(* Logix 5000 AddOnInstructionDefinition export; software revision 16.04 *)

ADD_ON_INSTRUCTION AMCI_ANG1E_Encoder_Follower   (* revision 1.1, vendor AMCI, ExecuteEnableInFalse *)
// Revision note:
// Version 1.1 added the slot_axis number and the input parameters can now be tags or discrete values.
VAR_INPUT
   Axis_Status_Bits : INT; {required}
   slot_axis_number : INT; {required}
   Electronic_Gearing_Numerator : INT; {required}
   Electronic_Gearing_Denominator : INT; {required}
   Programmed_Speed : DINT; {required}
   Acceleration : INT; {required}
   Deceleration : INT; {required}
   jerk : INT;
END_VAR
VAR_IN_OUT
   AMCI_ANG1E_output_data : INT[10]; {required}
END_VAR
VAR_OUTPUT
   EN : BOOL; {visible}
   Encoder_Follower_Occurring : BOOL; {visible}
   ER : BOOL; {visible}
END_VAR
VAR
   Upper_Result_X_1000 : DINT;
   command_data_block : INT[10];
        [0]   // Command Bits MSW
        [1]   // Command Bits LSW
        [4]   // Upper Programmed Speed
        [5]   // Lower Programmed Speed
   index : INT;
END_VAR

ROUTINE EnableInFalse   (* ladder *)
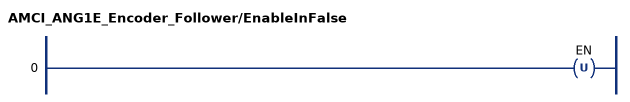
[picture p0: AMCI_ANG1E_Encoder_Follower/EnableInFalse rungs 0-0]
   0: OTU(EN);
END_ROUTINE

ROUTINE Logic   (* ladder *)
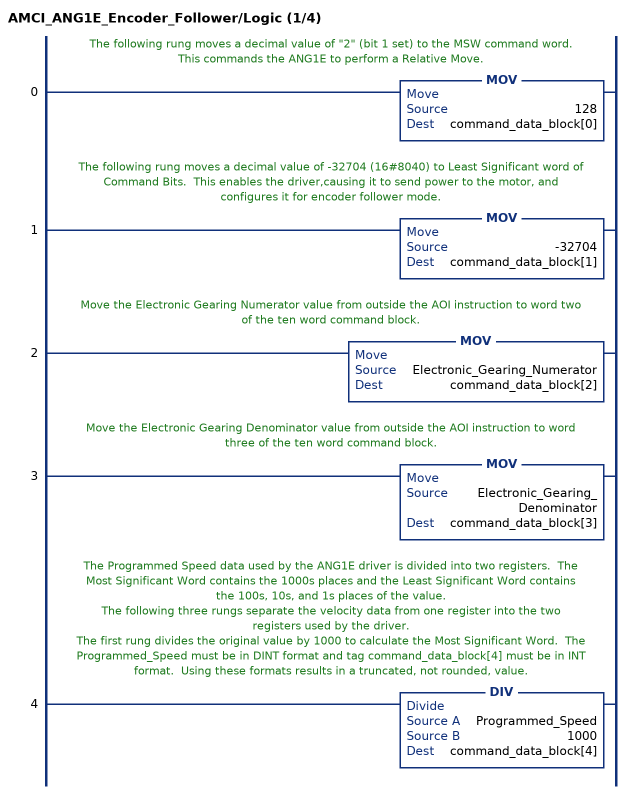
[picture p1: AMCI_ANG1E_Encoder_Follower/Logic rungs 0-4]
   // The following rung moves a decimal value of "2" (bit 1 set) to the MSW command word.  This commands the ANG1E to perform a Relative Move.
   0: MOV(128,command_data_block[0]);
   // The following rung moves a decimal value of -32704 (16#8040) to Least Significant word of Command Bits.  This enables the driver,causing it to send power to the motor, and configures it for encoder follower mode.
   1: MOV(-32704,command_data_block[1]);
   // Move the Electronic Gearing Numerator value from outside the AOI instruction to word two of the ten word command block.
   2: MOV(Electronic_Gearing_Numerator,command_data_block[2]);
   // Move the Electronic Gearing Denominator value from outside the AOI instruction to word three of the ten word command block.
   3: MOV(Electronic_Gearing_Denominator,command_data_block[3]);
   // The Programmed Speed data used by the ANG1E driver is divided into two registers.  The Most Significant Word contains the 1000s places and the Least Significant Word contains the 100s, 10s, and 1s places of the value.
   // The following three rungs separate the velocity data from one register into the two registers used by the driver.
   // The first rung divides the original value by 1000 to calculate the Most Significant Word.  The Programmed_Speed must be in DINT format and tag command_data_block[4] must be in INT format.  Using these formats results in a truncated, not rounded, value.
   4: DIV(Programmed_Speed,1000,command_data_block[4]);
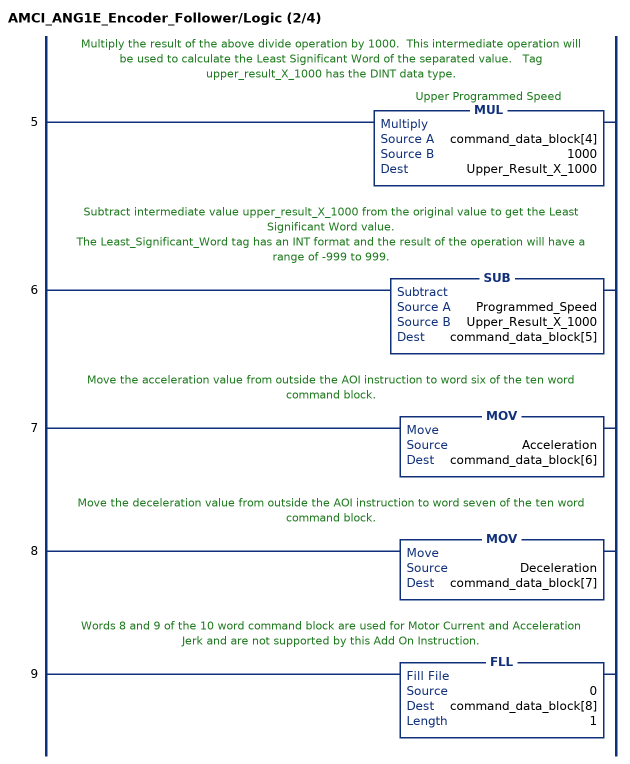
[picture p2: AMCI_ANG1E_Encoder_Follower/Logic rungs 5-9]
   // Multiply the result of the above divide operation by 1000.  This intermediate operation will be used to calculate the Least Significant Word of the separated value.   Tag upper_result_X_1000 has the DINT data type.
   5: MUL(command_data_block[4],1000,Upper_Result_X_1000);
   // Subtract intermediate value upper_result_X_1000 from the original value to get the Least Significant Word value.
   // The Least_Significant_Word tag has an INT format and the result of the operation will have a range of -999 to 999.
   6: SUB(Programmed_Speed,Upper_Result_X_1000,command_data_block[5]);
   // Move the acceleration value from outside the AOI instruction to word six of the ten word command block.
   7: MOV(Acceleration,command_data_block[6]);
   // Move the deceleration value from outside the AOI instruction to word seven of the ten word command block.
   8: MOV(Deceleration,command_data_block[7]);
   // Words 8 and 9 of the 10 word command block are used for Motor Current and Acceleration Jerk and are not supported by this Add On Instruction.
   9: FLL(0,command_data_block[8],1);
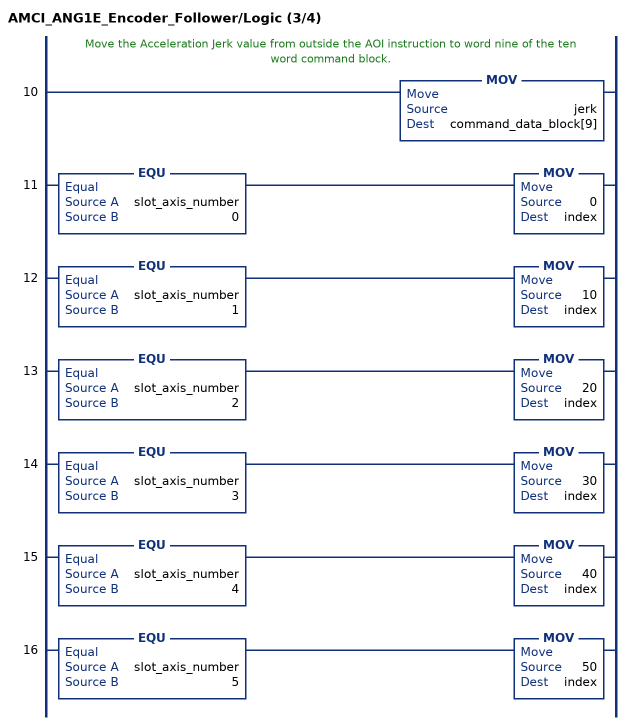
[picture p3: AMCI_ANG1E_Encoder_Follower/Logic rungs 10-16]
   // Move the Acceleration Jerk value from outside the AOI instruction to word nine of the ten word command block.
   10: MOV(jerk,command_data_block[9]);
   11: EQU(slot_axis_number,0)MOV(0,index);
   12: EQU(slot_axis_number,1)MOV(10,index);
   13: EQU(slot_axis_number,2)MOV(20,index);
   14: EQU(slot_axis_number,3)MOV(30,index);
   15: EQU(slot_axis_number,4)MOV(40,index);
   16: EQU(slot_axis_number,5)MOV(50,index);
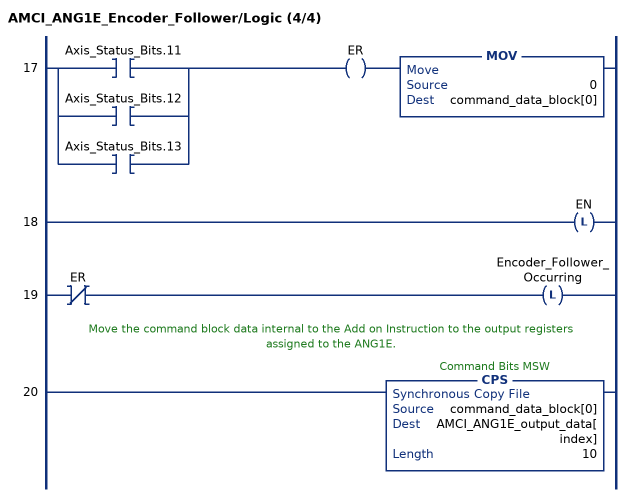
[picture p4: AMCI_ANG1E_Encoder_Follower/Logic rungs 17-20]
   17: [XIC(Axis_Status_Bits.11) ,XIC(Axis_Status_Bits.12) ,XIC(Axis_Status_Bits.13) ]OTE(ER)MOV(0,command_data_block[0]);
   18: OTL(EN);
   19: XIO(ER)OTL(Encoder_Follower_Occurring);
   // Move the command block data internal to the Add on Instruction to the output registers assigned to the ANG1E.
   20: CPS(command_data_block[0],AMCI_ANG1E_output_data[index],10);
END_ROUTINE
END_ADD_ON_INSTRUCTION
